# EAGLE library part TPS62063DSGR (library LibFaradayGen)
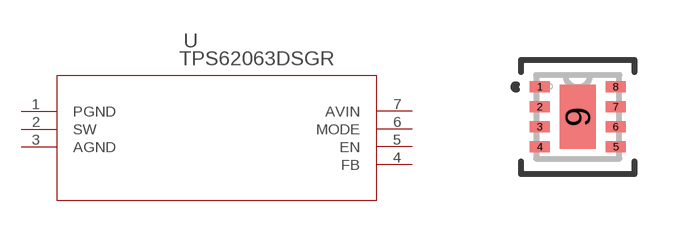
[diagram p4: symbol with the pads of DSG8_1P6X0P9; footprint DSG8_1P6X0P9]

Designator prefix U

## TPS62063DSGR (MANUFACTURER_PART_NUMBER: TPS62063DSGR; VENDOR: Texas Instruments)  [DSG8_1P6X0P9]
1  PGND  pwr
2  SW  out
3  AGND  in
4  FB  in
5  EN  in
6  MODE  in
7  AVIN  in

## Footprint DSG8_1P6X0P9 (pad centres in mm)
smd 0.5 x 0.28: 1 -0.95,0.75; 2 -0.95,0.25; 3 -0.95,-0.25; 4 -0.95,-0.75; 5 0.95,-0.75; 6 0.95,-0.25; 7 0.95,0.25; 8 0.95,0.75
smd 0.9 x 1.6: 9 0,0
